ORGANIZATION_BLOCK OB 1
BEGIN

	// Check instance-DB length
	AUF		DB 1
	L		DBLG
	__ASSERT==	__ACCU 1,	22
	AUF		DB 0


	//TODO
//	CALL	SFB 5, DB 1 (
//		IN	:= FALSE,
//		PT	:= T#0s,
//		Q	:= M 0.0,
//		ET	:= MD 2,
//	)
END_ORGANIZATION_BLOCK


DATA_BLOCK DB 1
	SFB 5
BEGIN
END_DATA_BLOCK
